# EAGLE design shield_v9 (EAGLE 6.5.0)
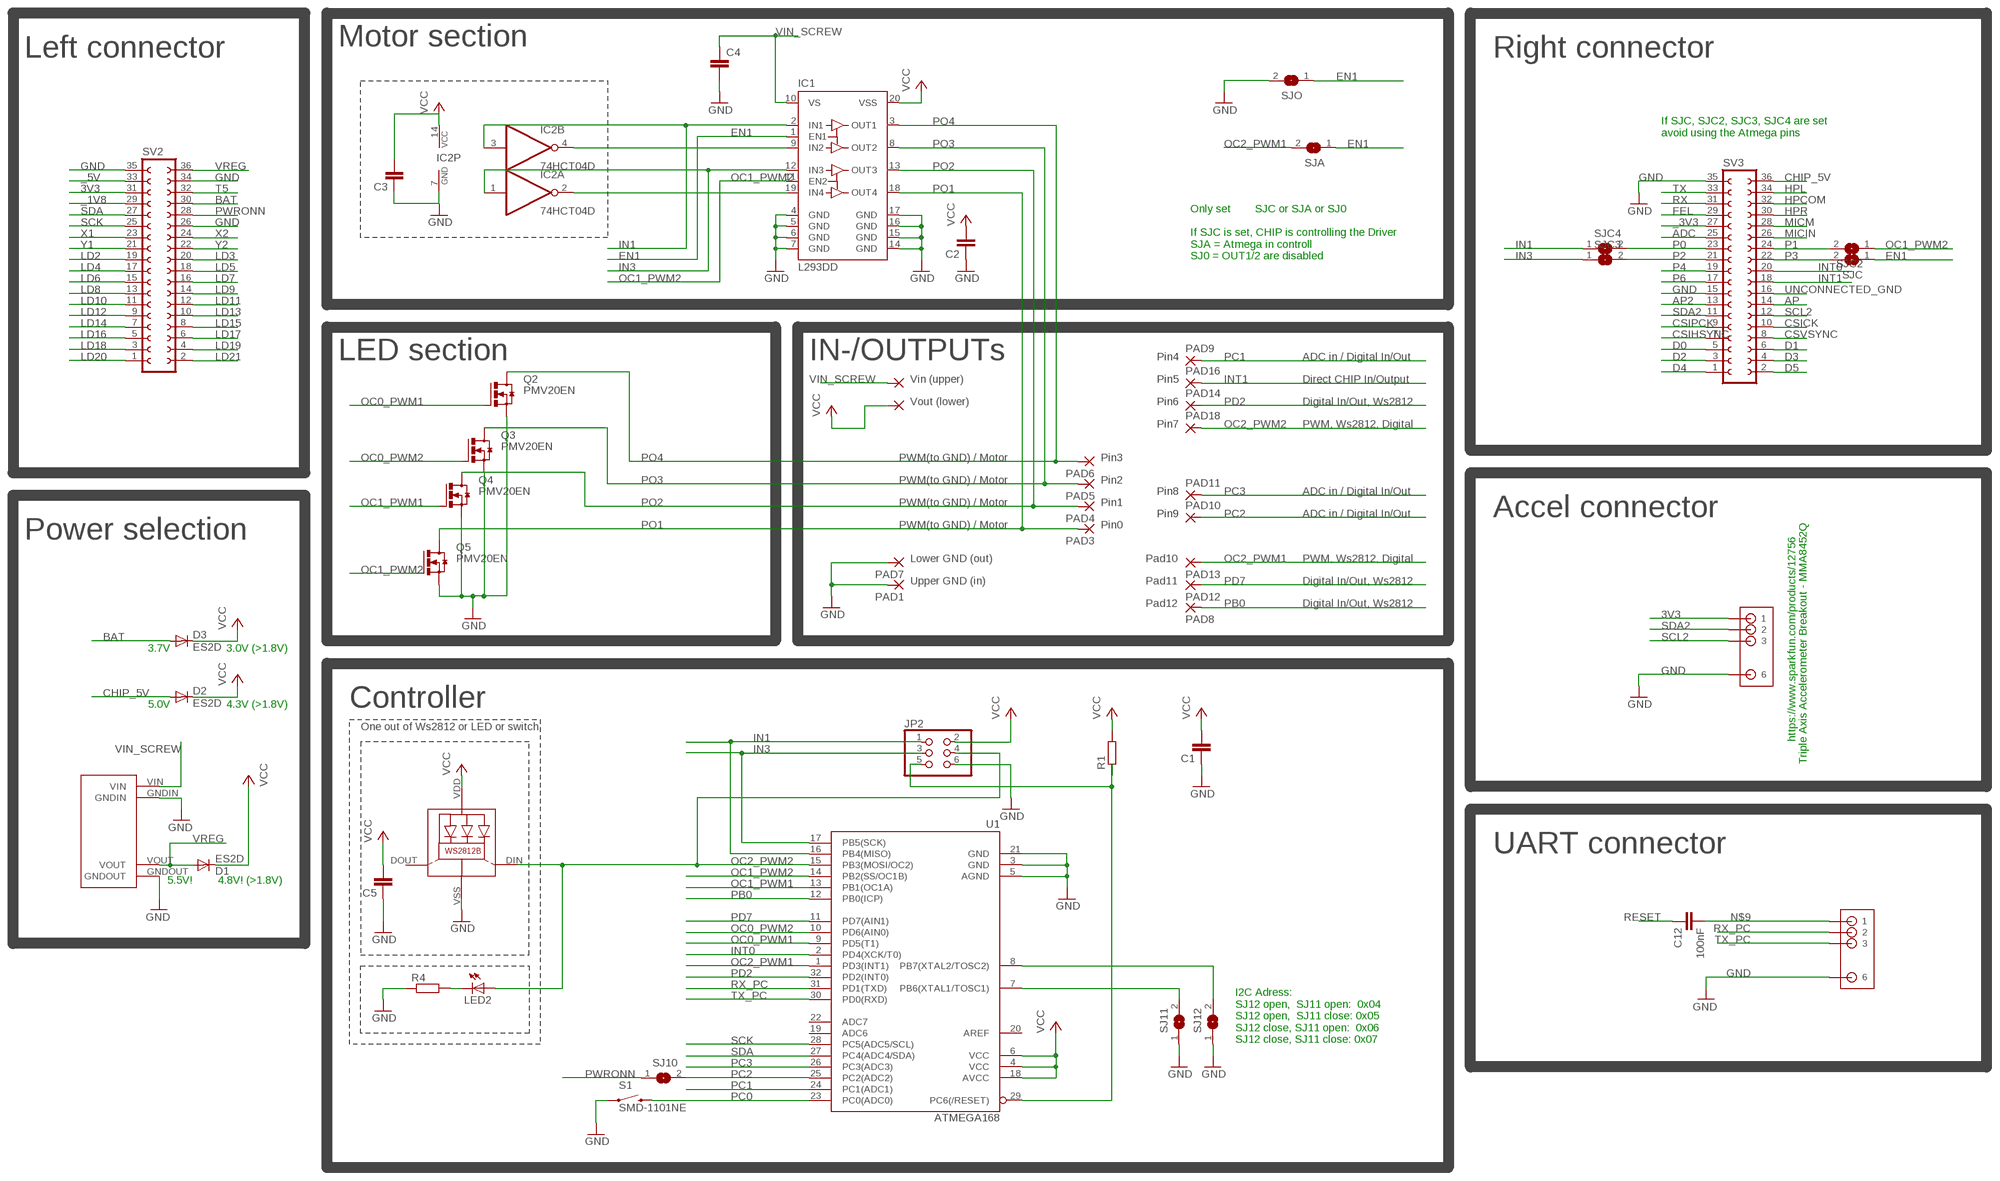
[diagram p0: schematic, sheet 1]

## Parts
C1  C-EUC0805  [C0805]
C2  C-EUC0805  [C0805]
C3  C-EUC0805  [C0805]
C4  C-EUC1210  [C1210]
C5  C-EUC0805  [C0805]
C12  100nF  C-EUC1206  [C1206]
D1  ES2D  [SMB]
D2  ES2D  [SMB]
D3  ES2D  [SMB]
IC1  L293DD  [SO20]
IC2  74HCT04D  [SO14]
JP2  PINHD-2X3  [2X03]
LED1  WS2812B  [WS2812B]
LED2  LEDCHIP-LED0805  [CHIP-LED0805]
PAD1  3,17/1,3  [3,17/1,3]
PAD2  3,17/1,3  [3,17/1,3]
PAD3  3,17/1,3  [3,17/1,3]
PAD4  3,17/1,3  [3,17/1,3]
PAD5  3,17/1,3  [3,17/1,3]
PAD6  3,17/1,3  [3,17/1,3]
PAD7  3,17/1,3  [3,17/1,3]
PAD8  WIREPADSMD1,27-254  [SMD1,27-2,54]
PAD9  3,17/1,3  [3,17/1,3]
PAD10  3,17/1,3  [3,17/1,3]
PAD11  3,17/1,3  [3,17/1,3]
PAD12  SMD2  [SMD1,27-2,54]
PAD13  SMD2  [SMD1,27-2,54]
PAD14  3,17/1,3  [3,17/1,3]
PAD16  3,17/1,3  [3,17/1,3]
PAD17  3,17/1,3  [3,17/1,3]
PAD18  3,17/1,3  [3,17/1,3]
Q2  PMV20EN  NMOSFET_SMD_223  [SOT223]
Q3  PMV20EN  NMOSFET_SMD_223  [SOT223]
Q4  PMV20EN  NMOSFET_SMD_223  [SOT223]
Q5  PMV20EN  NMOSFET_SMD_223  [SOT223]
R1  R-EU_M1206  [M1206]
R4  R-EU_M1206  [M1206]
S1  SMD-1101NE  SWITCH-MOMENTARY-2-SMD-1101NE  [TACTILE-SWITCH-1101NE]
SJ10  SJ  [SJ]
SJ11  SJ  [SJ]
SJ12  SJ  [SJ]
SJA  SJ  [SJ]
SJC  SJ  [SJ]
SJC2  SJ  [SJ]
SJC3  SJ  [SJ]
SJC4  SJ  [SJ]
SJO  SJ  [SJ]
SV2  FE18-2  [FE18-2]
SV3  FE18-2  [FE18-2]
U1  ATMEGA168  [TQFP32-08]
U$1  MP1584EN  [MP1584EN]
U$3  6_TO_4_HEADER  [6_TO_4_HEADER]
U$4  6_TO_4_HEADER  [6_TO_4_HEADER]

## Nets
3V3: SV2.31 U$4.1
_1V8: SV2.29
_3V3: SV3.27
_5V: SV2.33
ADC: SV3.25
AP: SV3.14
AP2: SV3.13
BAT: D3.A SV2.30
CHIP_5V: D2.A SV3.36
CSICK: SV3.10
CSIHSYNC: SV3.7
CSIPCK: SV3.9
CSVSYNC: SV3.8
D0: SV3.5
D1: SV3.6
D2: SV3.3
D3: SV3.4
D4: SV3.1
D5: SV3.2
EN1: IC1.1(EN1) SJA.1 SJC.1 SJO.1
FEL: SV3.29
GND: C1.1 C2.1 C3.1 C4.2 C5.1 IC1.4(GND) IC1.5(GND) IC1.6(GND) IC1.7(GND) IC1.14(GND) IC1.15(GND) IC1.16(GND) IC1.17(GND) IC2.7(P:GND) JP2.6 LED1.VSS(GND) PAD1.1(P) PAD7.1(P) Q2.3(S) Q3.3(S) Q4.3(S) Q5.3(S) R4.1 S1.P$1 SJ11.1 SJ12.1 SJO.2 SV2.26 SV2.34 SV2.35 SV3.15 SV3.35 U1.3(GND) U1.5(AGND) U1.21(GND) U$1.GNDIN U$1.GNDOUT U$3.6 U$4.6
HPCOM: SV3.32
HPL: SV3.34
HPR: SV3.30
IN1: IC1.2(IN1) IC2.3(B:I) JP2.1 SJC4.1 U1.16(PB4(MISO))
IN3: IC1.12(IN3) IC2.1(A:I) JP2.3 SJC3.1 U1.17(PB5(SCK))
INT0: SV3.20 U1.2(PD4(XCK/T0))
INT1: PAD16.1(P) SV3.18
LD2: SV2.19
LD3: SV2.20
LD4: SV2.17
LD5: SV2.18
LD6: SV2.15
LD7: SV2.16
LD8: SV2.13
LD9: SV2.14
LD10: SV2.11
LD11: SV2.12
LD12: SV2.9
LD13: SV2.10
LD14: SV2.7
LD15: SV2.8
LD16: SV2.5
LD17: SV2.6
LD18: SV2.3
LD19: SV2.4
LD20: SV2.1
LD21: SV2.2
MICIN: SV3.26
MICM: SV3.28
N$1: IC1.19(IN4) IC2.2(A:O)
N$2: SJ11.2 U1.7(PB6(XTAL1/TOSC1))
N$3: SJ12.2 U1.8(PB7(XTAL2/TOSC2))
N$4: LED2.C R4.2
N$9: C12.2 U$3.1
N$11: IC1.9(IN2) IC2.4(B:O)
OC0_PWM1: Q2.1(G) U1.9(PD5(T1))
OC0_PWM2: Q3.1(G) U1.10(PD6(AIN0))
OC1_PWM1: Q4.1(G) U1.13(PB1(OC1A))
OC1_PWM2: IC1.11(EN2) Q5.1(G) SJC2.1 U1.14(PB2(SS/OC1B))
OC2_PWM1: PAD13.1(P) SJA.2 U1.1(PD3(INT1))
OC2_PWM2: JP2.4 LED1.DIN(DI) LED2.A PAD18.1(P) U1.15(PB3(MOSI/OC2))
P0: SJC4.2 SV3.23
P1: SJC2.2 SV3.24
P2: SJC3.2 SV3.21
P3: SJC.2 SV3.22
P4: SV3.19
P6: SV3.17
PB0: PAD8.1(P) U1.12(PB0(ICP))
PC0: S1.P$2 U1.23(PC0(ADC0))
PC1: PAD9.1(P) U1.24(PC1(ADC1))
PC2: PAD10.1(P) SJ10.2 U1.25(PC2(ADC2))
PC3: PAD11.1(P) U1.26(PC3(ADC3))
PD2: PAD14.1(P) U1.32(PD2(INT0))
PD7: PAD12.1(P) U1.11(PD7(AIN1))
PO1: IC1.18(OUT4) PAD3.1(P) Q5.2(D) Q5.4(D)
PO2: IC1.13(OUT3) PAD4.1(P) Q4.2(D) Q4.4(D)
PO3: IC1.8(OUT2) PAD5.1(P) Q3.2(D) Q3.4(D)
PO4: IC1.3(OUT1) PAD6.1(P) Q2.2(D) Q2.4(D)
PWRONN: SJ10.1 SV2.28
RESET: C12.1 JP2.5 R1.1 U1.29(PC6(/RESET))
RX: SV3.31
RX_PC: U1.31(PD1(TXD)) U$3.2
SCK: SV2.25 U1.28(PC5(ADC5/SCL))
SCL2: SV3.12 U$4.3
SDA: SV2.27 U1.27(PC4(ADC4/SDA))
SDA2: SV3.11 U$4.2
T5: SV2.32
TX: SV3.33
TX_PC: U1.30(PD0(RXD)) U$3.3
UNCONNECTED_GND: SV3.16
VCC: C1.2 C2.2 C3.2 C5.2 D1.C D2.C D3.C IC1.20(VSS) IC2.14(P:VCC) JP2.2 LED1.VDD PAD17.1(P) R1.2 U1.4(VCC) U1.6(VCC) U1.18(AVCC)
VIN_SCREW: C4.1 IC1.10(VS) PAD2.1(P) U$1.VIN
VREG: D1.A SV2.36 U$1.VOUT
X1: SV2.23
X2: SV2.24
Y1: SV2.21
Y2: SV2.22
Unconnected: IC2.5(C:I) IC2.6(C:O) IC2.8(D:O) IC2.9(D:I) IC2.10(E:O) IC2.11(E:I) IC2.12(F:O) IC2.13(F:I) LED1.DOUT(DO) U1.19(ADC6) U1.20(AREF) U1.22(ADC7)

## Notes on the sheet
- Motor section
- Left connector | Right connector
- If SJC, SJC2, SJC3, SJC4 are set 
  avoid using the Atmega pins
- Only set        SJC or SJA or SJ0
  
  If SJC is set, CHIP is controlling the Driver
  SJA = Atmega in controll
  SJ0 = OUT1/2 are disabled
- LED section | IN-/OUTPUTs | Pin4 | ADC in / Digital In/Out
- Vin (upper) | Pin5 | Direct CHIP In/Output
- Vout (lower) | Pin6 | Digital In/Out, Ws2812
- Pin7 | PWM, Ws2812, Digital
- PWM(to GND) / Motor | Pin3
- PWM(to GND) / Motor | Pin2
- Pin8 | ADC in / Digital In/Out
- PWM(to GND) / Motor | Pin1
- Pin9 | ADC in / Digital In/Out | Accel connector
- PWM(to GND) / Motor | Pin0
- Power selection
- Lower GND (out) | Pad10 | PWM, Ws2812, Digital
- Upper GND (in) | Pad11 | Digital In/Out, Ws2812
- Pad12 | Digital In/Out, Ws2812
- 3.7V | 3.0V (>1.8V)
- 5.0V | 4.3V (>1.8V) | Controller
- One out of Ws2812 or LED or switch
- https://www.sparkfun.com/products/12756
- Triple Axis Accelerometer Breakout - MMA8452Q
- UART connector
- 5.5V! | 4.8V! (>1.8V)
- I2C Adress: 
  SJ12 open,  SJ11 open:  0x04
  SJ12 open,  SJ11 close: 0x05
  SJ12 close, SJ11 open:  0x06
  SJ12 close, SJ11 close: 0x07

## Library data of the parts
C1-C5 C12 = rcl:C-EU: CAPACITOR, European symbol
D1-D3 = diode:ES2D: DIODE
IC1 = st-microelectronics:L293DD: PUSH-PULL FOUR CHANNEL DRIVER WITH DIODES Source: http://www.st.com/stonline/books/pdf/docs/1330.pdf; OC_FARNELL: unknown
IC2 = 74xx-eu:74*04: Hex INVERTER
JP2 = pinhead:PINHD-2X3: PIN HEADER
LED1 = WS2812B:WS2812B: Features and Benefits  * Intelligent reverse connect protection, the power supply reverse connection does not damage the IC. * The control circuit and the LED share the only power source. Control circuit and RGB chip are integrated in a package of 5050 components, form a complete control of pixel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
LED2 = led:LED: LED
PAD1-PAD7 PAD9-PAD11 PAD14 PAD16-PAD18 = wirepad:3,17/1,3: THROUGH-HOLE PAD
PAD8 = wirepad:WIREPAD: Wire PAD connect wire on PCB
PAD12 PAD13 = wirepad:SMD2: SMD PAD
Q2-Q5 = transistor-power:NMOSFET_SMD_223
R1 R4 = rcl:R-EU_: RESISTOR, European symbol
S1 = SparkFun-Electromechanical:SWITCH-MOMENTARY-2: Various NO switches- pushbuttons, reed, etc
SJ10-SJ12 SJA SJC SJC2-SJC4 SJO = jumper:SJ: SMD solder JUMPER
SV2 SV3 = con-lsta:FE18-2: FEMALE HEADER; OC_FARNELL: unknown; OC_NEWARK: unknown
U1 = SparkFun-DigitalIC:ATMEGA168: Atmel 32-pin 8-bit micro, 16k flash.
U$1 = power_supply:MP1584EN
U$3 U$4 = power_supply:6_TO_4_HEADER

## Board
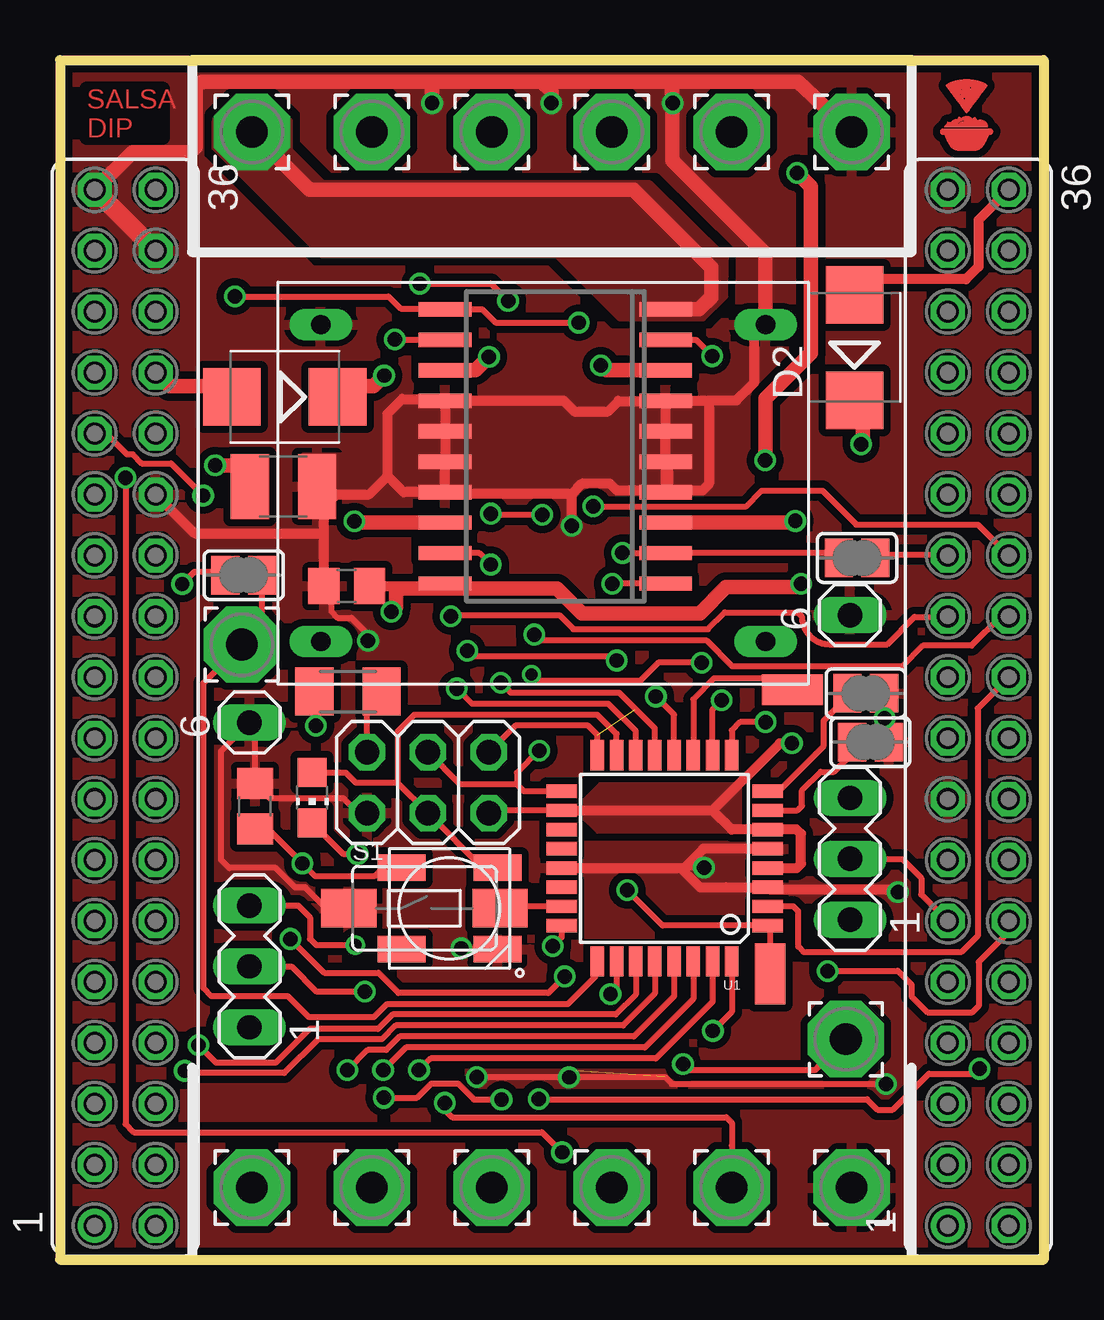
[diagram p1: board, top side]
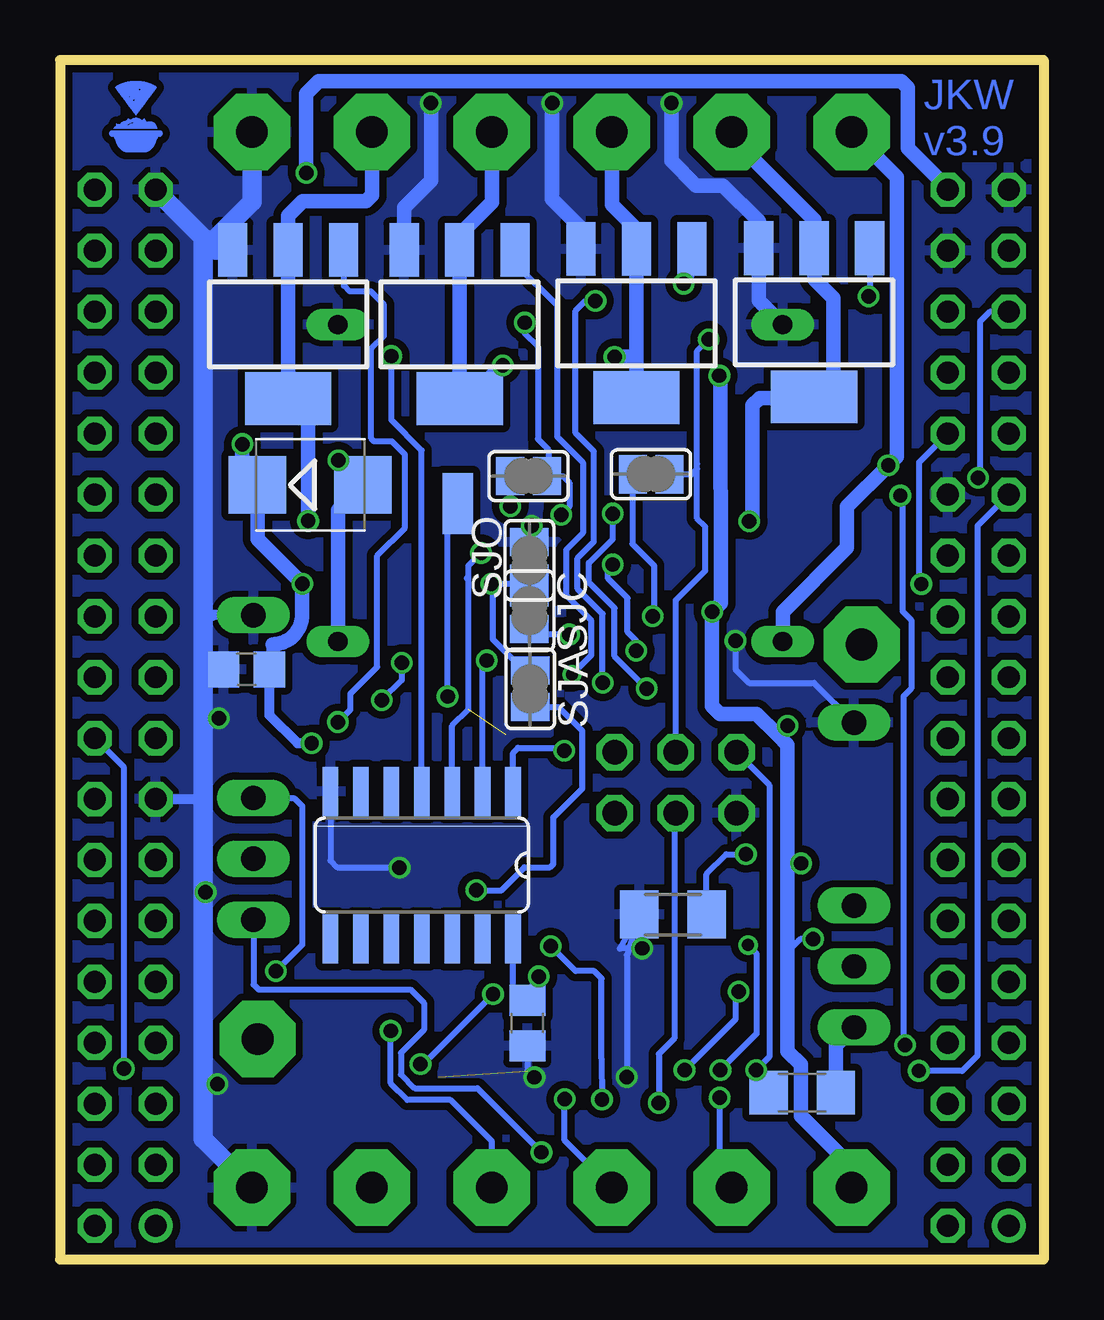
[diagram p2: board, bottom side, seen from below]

Size 41 x 50 mm. Coordinates in mm from the lower left corner, seen from the top.
Outline: 0,50 41,50 41,0 0,0 0,50
Copper layers (1*16): Top 0.035mm / dielectric 1.5mm / Bottom 0.035mm
Design rules "SeeedStudio_2layer_DRU_no_angle_20140221": minimum track width 6mil, minimum drill 12mil, track to track 6mil, track to pad 6mil, pad to pad 6mil, via to via 6mil, smd to smd 0mil, copper to edge 10mil, drill to drill 10mil, minimum pad ring 10mil, minimum via ring 6mil, stop-mask expansion 2mil, vias tented up to drill 100mil, thermal gap 10mil

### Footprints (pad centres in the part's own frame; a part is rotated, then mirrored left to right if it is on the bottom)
C0805 = smd 1.3 x 1.5: 1 -0.95,0; 2 0.95,0
C1210 = smd 1.6 x 2.7: 1 -1.4,0; 2 1.4,0
C1206 = smd 1.6 x 1.8: 1 -1.4,0; 2 1.4,0
SMB = smd 2.4 x 2.4: A 2.2,0; C -2.2,0
SO20 = smd 0.6 x 2.2: 1 -5.715,-4.6; 2 -4.445,-4.6; 3 -3.175,-4.6; 4 -1.905,-4.6; 5 -0.635,-4.6; 6 0.635,-4.6; 7 1.905,-4.6; 8 3.175,-4.6; 9 4.445,-4.6; 10 5.715,-4.6; 11 5.715,4.6; 12 4.445,4.6; 13 3.175,4.6; 14 1.905,4.6; 15 0.635,4.6; 16 -0.635,4.6; 17 -1.905,4.6; 18 -3.175,4.6; 19 -4.445,4.6; 20 -5.715,4.6
SO14 = smd 0.66 x 2.032: 1 -3.81,-3.073; 2 -2.54,-3.073; 3 -1.27,-3.073; 4 0,-3.073; 5 1.27,-3.073; 6 2.54,-3.073; 7 3.81,-3.073; 8 3.81,3.073; 9 2.54,3.073; 10 1.27,3.073; 11 0,3.073; 12 -1.27,3.073; 13 -2.54,3.073; 14 -3.81,3.073
2X03 = drill 1.016 octagon: 1 -2.54,-1.27; 2 -2.54,1.27; 3 0,-1.27; 4 0,1.27; 5 2.54,-1.27; 6 2.54,1.27
WS2812B = smd 2 x 1.1: DIN 2,1.7; DOUT -2,-1.7; VDD -2,1.7; VSS 2,-1.7
CHIP-LED0805 = smd 1.2 x 1.2: A 0,-1.05; C 0,1.05
3,17/1,3 = drill 1.321 pad 3.175 octagon: 1 0,0
SMD1,27-2,54 = smd 1.27 x 2.54: 1 0,0
SOT223 = smd 1.219 x 2.235: 1 -2.311,-3.099; 2 0,-3.099; 3 2.311,-3.099 | smd 3.6 x 2.2: 4 0,3.099
M1206 = smd 1.6 x 2: 1 -1.4,0; 2 1.4,0
TACTILE-SWITCH-1101NE = smd 2.3 x 1.6: P$1 -3.15,0; P$2 3.15,0
SJ = smd 1.168 x 1.6: 1 -0.762,0; 2 0.762,0
FE18-2 = drill 0.914: 1 -21.59,1.27 | drill 0.914 octagon: 2 -21.59,-1.27; 3 -19.05,1.27; 4 -19.05,-1.27; 5 -16.51,1.27; 6 -16.51,-1.27; 7 -13.97,1.27; 8 -13.97,-1.27; 9 -11.43,1.27; 10 -11.43,-1.27; 11 -8.89,1.27; 12 -8.89,-1.27; 13 -6.35,1.27; 14 -6.35,-1.27; 15 -3.81,1.27; 16 -3.81,-1.27; 17 -1.27,1.27; 18 -1.27,-1.27; 19 1.27,1.27; 20 1.27,-1.27; 21 3.81,1.27; 22 3.81,-1.27; 23 6.35,1.27; 24 6.35,-1.27; 25 8.89,1.27; 26 8.89,-1.27; 27 11.43,1.27; 28 11.43,-1.27; 29 13.97,1.27; 30 13.97,-1.27; 31 16.51,1.27; 32 16.51,-1.27; 33 19.05,1.27; 34 19.05,-1.27; 35 21.59,1.27; 36 21.59,-1.27
TQFP32-08 = smd 1.27 x 0.559: 1 -4.293,2.8; 2 -4.293,2; 3 -4.293,1.2; 4 -4.293,0.4; 5 -4.293,-0.4; 6 -4.293,-1.2; 7 -4.293,-2; 8 -4.293,-2.8; 17 4.293,-2.8; 18 4.293,-2; 19 4.293,-1.2; 20 4.293,-0.4; 21 4.293,0.4; 22 4.293,1.2; 23 4.293,2; 24 4.293,2.8 | smd 0.559 x 1.27: 9 -2.8,-4.293; 10 -2,-4.293; 11 -1.2,-4.293; 12 -0.4,-4.293; 13 0.4,-4.293; 14 1.2,-4.293; 15 2,-4.293; 16 2.8,-4.293; 25 2.8,4.293; 26 2,4.293; 27 1.2,4.293; 28 0.4,4.293; 29 -0.4,4.293; 30 -1.2,4.293; 31 -2,4.293; 32 -2.8,4.293
MP1584EN = drill 0.8 long: GNDIN 1.778,14.986; GNDOUT 20.32,14.986; VIN 1.778,1.778; VOUT 20.32,1.778
6_TO_4_HEADER = drill 1.016 long: 1 0,-6.35; 2 0,-3.81; 3 0,-1.27; 6 0,6.35

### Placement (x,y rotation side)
C1  33.22,24.6 0 bottom
C2  11.95,28.07 0 top
C3  21.52,9.85 90 bottom
C4  9.32,32.22 0 top
C5  8.13,18.9 270 top
C12  10.06,6.96 0 bottom
D1  30.57,32.28 0 bottom
D2  33.12,38.01 90 top
D3  9.37,35.95 180 top
IC1  20.65,33.89 90 top
IC2  25.92,16.44 180 bottom
JP2  15.34,19.88 180 top
LED1  16.23,14.63 0 top
LED2  10.52,19.25 180 top
PAD1  33,47 0 top
PAD2  8,47 0 top
PAD3  13,47 0 top
PAD4  18,47 0 top
PAD5  23,47 0 top
PAD6  28,47 0 top
PAD7  33,3 0 top
PAD8  24.42,31.5 180 bottom
PAD9  13,3 0 top
PAD10  7.58,25.63 0 top
PAD11  32.76,9.18 0 top
PAD12  30.52,23.76 270 top
PAD13  29.6,11.9 180 top
PAD14  23,3 0 top
PAD16  18,3 0 top
PAD17  8,3 0 top
PAD18  28,3 0 top
Q2  31.49,38.98 180 bottom
Q3  24.34,38.98 180 bottom
Q4  16.97,39.02 180 bottom
Q5  9.56,39.06 180 bottom
R1  12.01,23.67 180 top
R4  15.45,14.38 0 bottom
S1  15.19,14.64 0 top
SJ10  7.66,28.52 0 top
SJ11  33.78,21.56 180 top
SJ12  33.59,23.6 180 top
SJA  21.4,23.79 270 bottom
SJC  21.43,27.05 270 bottom
SJC2  21.47,32.66 180 bottom
SJC3  16.36,32.74 180 bottom
SJC4  33.23,29.24 0 top
SJO  21.43,29.15 90 bottom
SV2  2.72,23 90 top
SV3  38.28,23 90 top
U1  25.2,16.72 180 top
U$1  9.09,23.98 0 top
U$2  LOGO  [LOGO]  36.54,46.02 0 top
U$3  7.9,16.03 0 top
U$4  32.93,20.51 0 top
U$5  LOGO  [LOGO]  39.09,46.1 0 bottom

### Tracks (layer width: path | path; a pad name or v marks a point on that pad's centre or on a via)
3V3  (via drill 0.6)
  Top 0.254: v2.73,32.59 2.73,5.65 3.07,5.31 20.09,5.31 v20.93,4.47
  Bottom 0.254: U$4.1 32.93,11.47 32.72,11.25 26.39,11.25 25.83,10.69 25.83,9.56 26.78,8.61 26.78,7.71 26.21,7.14 23.6,7.14 v20.93,4.47 | SV2.31 2.23,39.51 2.65,39.09 2.65,32.66 v2.73,32.59
BAT
  Top 0.61: SV2.30 4.56,36.4 6.73,36.4 D3.A
CHIP_5V
  Top 0.406: SV3.36 38.29,43.33 38.29,41.38 37.77,40.86 34.13,40.86 D2.A
EN1  (via drill 0.6)
  Top 0.254: IC1.1 v23.03,28.18 v23.02,28.17
  Bottom 0.254: SJA.1 21.65,24.55 22.95,25.84 22.95,28.09 v23.02,28.17 21.65,28.17 SJO.1 SJC.1 21.2,28.18
  Bottom 0.406: 21.37,27.87 SJC.1
GND  (via drill 0.6)  (1 unrouted)
  Top 0.254: C5.1 8.13,22.15 U$3.6 6.72,21.2 6.72,16.66 7.06,16.32 8.99,16.32 9.79,15.52 10.22,15.52 11.1,14.64 S1.P$1 | v26.85,16.33 26.18,16.33 26.11,16.4 | 34.35,21.75 SJ11.1 34.38,21.73 v34.38,22.57 34.35,22.59 SJ12.1 | C2.1 11.3,27.77 11.3,27.03 11.58,26.75 12.15,26.75 12.84,26.06 v12.84,25.79 | LED1.VSS 16.76,12.93 v16.73,12.97 | v17.37,7.61 25.21,7.61 25.5,7.32 v34.44,7.32 | C5.1 | JP2.6 12.43,18.61 11.82,19.21 8.76,19.21 C5.1
  Top 0.406: U1.21 25.87,16.32 25.95,16.24 | 29.45,17.08 U1.5 26.82,17.12 26.11,16.4 25.95,16.24 | 27.77,15.52 U1.3 | 25.95,16.24 26.67,15.52 U1.3 | IC1.7 23.28,35.79 22.84,35.34 21.45,35.34 21,35.8 IC1.14 IC1.15 | IC1.7 27.03,35.8 27.05,35.81 | 27.05,35.81 27.05,32.32 26.78,32.05 25.32,32.05 | 25.32,32.05 IC1.4 | 25.32,32.05 23.22,32.05 22.94,32.33 21.77,32.33 21.35,31.91 | 21.35,31.91 16.12,31.91 IC1.17 | IC1.17 14.33,31.99 13.65,32.66 | 13.65,32.66 13.65,35.26 14.26,35.87 16,35.87 16.03,35.84 | 27.05,35.81 28.21,35.81 28.94,36.55 28.94,38.49 U$1.GNDOUT | IC1.17 IC1.16 | IC1.15 16.05,33.28 16.07,33.26 16.07,34.51 IC1.15 | IC1.7 25.24,32.09 25.38,31.95 25.38,33.13 IC1.5 IC1.6 | 13.65,32.66 12.88,31.89 11.53,31.89 11,31.36 11,30.26 | C2.1 11,30.26 | SV2.26 5.62,30.26 11,30.26 | U1.3 29.58,15.43 34.81,15.43 v34.93,15.31 | SJ11.1 34.51,21.6 | v21.34,30.58 21.34,31.9 21.35,31.91
  Top 0.61: 15.51,49.1 20.08,49.1 | 20.08,49.1 25.51,49.1 | 25.51,49.1 30.77,49.1 PAD1.1 | 25.51,49.1 25.51,48.52 v25.54,48.2 25.54,45.8 29.41,41.92 U$1.GNDOUT | v15.51,48.2 15.51,49.1 | v20.48,48.2 20.48,48.7 20.08,49.1 | 15.51,49.1 5.92,49.1 5.66,48.84 5.66,46.35 5.47,46.16 3.02,46.16 SV2.35
  Top 0.813: SV2.35 SV2.34
  Bottom 0.254: R4.1 17.37,12.68 v17.37,7.61 | 17.65,12.95 R4.1 | C3.1 21.52,7.87 v21.22,7.59 | 34.63,26.84 35.04,27.24 | IC2.7 29.73,16.63 29.44,16.34 26.86,16.34 v26.85,16.33 | C1.1 34.26,24.69 35.04,24.69 | 32.63,47.37 PAD1.1 | v12.84,25.79 12.84,24.6 12.28,24.04 9.56,24.04 U$3.6 | v16.73,12.97 17.66,12.97 R4.1
  Bottom 0.406: SV3.15 35.11,19.19 35.04,19.12 | 35.05,15.41 35.04,15.42 | 35.04,15.2 v34.93,15.31 34.93,15.71 35.04,15.82 | 35,21.45 35.04,21.41 | 34.92,21.43 34.9,21.45 35.04,21.59 35.04,21.61 | 34.89,26.55 35.04,26.4 | v34.44,7.32 35.04,7.32 | 34.84,38.95 35.04,38.75 | v34.38,22.57 34.56,22.49 35.04,22.02 | U$4.6 34.61,26.86 34.63,26.84 | SJO.2 21.37,30.54 v21.34,30.58
  Bottom 0.61: Q3.3 26.65,43.85 25.54,44.96 v25.54,48.2 | v15.51,48.2 15.51,45.8 14.48,44.77 13.36,44.77 11.87,43.28 Q5.3 11.87,39.96 U$1.GNDIN | Q4.3 19.28,42.99 20.49,44.2 20.48,44.21 v20.48,48.2
  Bottom 0.813: 35.04,42.6 35.04,38.75 35.04,27.24 35.04,26.4 35.04,24.69 35.04,22.02 35.04,21.61 35.04,21.41 35.04,19.12 35.04,15.82 35.04,15.42 35.04,15.2 35.04,7.32 35.04,5.04 PAD7.1 | Q2.3 34.52,42.08 34.76,42.33 | 34.76,42.33 35.04,42.6 | PAD1.1 33,44.09 34.76,42.33 | SV3.35 37.01,44.57 35.04,42.6
  pour Top (isolate 0.305, rank 2): -0.07,0.25 40.88,0.25 41.01,10.57 41.01,50.01 0,50.01 0,10.47
  pour Bottom (isolate 0.305): 0,50 41.05,50 41.05,0.25 0.02,0.25 0.02,49.92
  pour Top (isolate 0.305, no thermals): 13.28,33.52 14.05,35.84 20.97,35.9 21.42,35.45 22.83,35.45 23.2,35.81 28.13,35.81 28.24,35.7 28.24,32.35 27.85,31.95 23.33,31.95 23.05,32.23 21.77,32.23 21.4,31.86 11.16,31.85 10.36,32.65 10.15,33.49
IN1  (via drill 0.6)  (1 unrouted)
  Top 0.254: JP2.1 18.98,22.25 22.02,22.25 22.4,21.87 U1.16 | v23.44,29.45 IC1.2 32.26,29.45 SJC4.1
  Bottom 0.254: IC2.3 24.65,22.25 23.98,22.92 23.98,28.46 | 23.98,28.46 23.98,28.92 v23.44,29.45 | 24.04,28.4 23.98,28.46
IN3  (via drill 0.6)
  Top 0.254: U1.17 19.34,19.52 19.05,19.81 | 19.05,19.81 16.68,19.81 JP2.3 | v19.98,21.21 19.05,20.28 19.05,19.81 | v13.96,38.35 16.03,38.35 IC1.12
  Bottom 0.254: JP2.3 15.34,27.47 14.1,28.71 14.1,30.54 14.44,30.89 14.44,32.96 | IC2.1 22.11,21.12 21.91,21.32 20.09,21.32 v19.98,21.21 | 14.22,38.09 v13.96,38.35 14.44,37.87 14.44,33.16 14.44,32.96 | SJC3.1 14.66,32.73 14.44,32.96
INT0
  Top 0.254: SV3.20 38.25,22.97 38.25,13.49 37.59,12.83 30.99,12.83 30.77,13.04 30.77,14.52 30.57,14.72 U1.2
INT1  (via drill 0.6)
  Top 0.254: v38.33,7.95 38.13,7.75 36.22,7.75 34.72,6.25 34.07,6.25 33.64,6.68 v19.96,6.68
  Bottom 0.254: PAD16.1 19.96,4.96 v19.96,6.68 | v38.33,7.95 38.33,20.51 SV3.18
N$1  (via drill 0.6)
  Top 0.254: 17.21,25.15 v16.98,25.38 17.22,25.13 23.04,25.13 v23.2,24.97 | v17.96,28.97 17.48,29.45 IC1.19
  Bottom 0.254: IC2.2 23.38,24.83 23.34,24.83 v23.2,24.97 | v16.98,25.38 16.98,25.79 17.34,26.15 17.34,27.57 18.15,28.38 18.15,28.78 v17.96,28.97
N$2
  Top 0.254: U1.7 30.75,18.72 30.94,18.91 30.94,19.56 31.71,20.33 32.27,20.33 33.03,21.09 33.03,21.78 33.03,22.12
  Top 0.406: SJ11.2 33.03,21.58 33.03,21.78
N$3
  Top 0.254: U1.8 29.95,19.52 31.84,21.41 31.84,22.47 32.83,23.46 SJ12.2
N$4  (via drill 0.6)
  Top 0.254: LED2.C 11.82,16.89 v12.41,16.89
  Bottom 0.254: R4.2 14.05,16.06 13.22,16.89 v12.41,16.89
N$9
  Bottom 0.406: 7.9,9.61 U$3.1
  Bottom 0.61: C12.2 8.66,8.92 U$3.1
N$11  (via drill 0.6)
  Top 0.254: IC1.9 26.51,38.34 v27.19,37.66
  Bottom 0.254: IC2.4 25.92,33.73 27.19,35 v27.19,37.66
OC0_PWM1  (via drill 0.6)
  Top 0.254: v29.41,22.4 28.35,22.4 28,22.06 U1.9
  Bottom 0.254: v29.41,22.4 28.89,22.93 28.89,23.59 27.77,24.7 27.77,29.34 26.62,30.49 26.62,33.55 27.16,34.1 27.9,34.1 28.03,34.23 28.03,37.96 27.5,38.49 27.5,39.8 28.04,40.35 28.92,40.35 29.16,40.59 29.16,41.4 29.18,41.42 | 29.13,42.03 Q2.1
  Bottom 0.406: 29.18,41.42 Q2.1
OC0_PWM2  (via drill 0.5, 0.6)
  Top 0.254: U1.10 27.2,22.93 v27.58,23.32 | v19.66,24.38 19.91,24.13 24.19,24.13 24.94,24.88 v26.75,24.88
  Bottom 0.254: 22.1,42.01 Q3.1 22.03,41.51 20.27,39.75 20.27,34.29 19.2,33.22 19.2,30.28 19.89,29.59 19.89,27.67 18.85,26.63 18.85,25.2 v19.66,24.38 | v27.58,23.32 26.75,24.16 v26.75,24.88
  Bottom 0.406: Q3.1 22.06,42.05
OC1_PWM1  (via drill 0.6)
  Top 0.254: U1.13 24.8,22.14 23.32,23.62 18.8,23.62 v18.38,24.04 | v15,40.68 17.96,40.68 v18.68,39.96
  Bottom 0.254: v18.68,39.96 19.09,39.96 19.51,39.54 19.51,34.44 18.75,33.68 18.75,29.92 19.42,29.25 19.42,27.95 18.38,26.91 v18.38,24.04 | Q4.1 14.66,41.02 v15,40.68
OC1_PWM2  (via drill 0.6)
  Top 0.254: U1.14 24,22.02 22.86,23.16 17.18,23.16 v16.54,23.8 | v7.29,40.15 13.69,40.15 14.2,39.64 16.02,39.64 IC1.11 17.59,39.61 18.15,39.05 v21.63,39.05 | v20.1,31.04 18.01,31.04 v17.96,31.09
  Bottom 0.254: v16.54,23.8 17.88,25.14 17.88,27.15 18.95,28.22 18.95,29.03 17.96,30.02 v17.96,31.09 17.88,31.01 | Q5.1 7.25,40.19 v7.29,40.15 | v21.63,39.05 21.63,38.59 21.08,38.05 21.08,34.2 20.64,33.76 20.64,32.72 SJC2.1 20.03,32.66 19.76,32.38 19.76,31.38 v20.1,31.04
  Bottom 0.406: 7.25,42.99 Q5.1
OC2_PWM1  (via drill 0.6)
  Top 0.254: v23.65,15.39 25.12,13.92 U1.1 29.6,13.81 PAD13.1
  Bottom 0.254: v23.65,15.39 22.59,15.39 21.64,16.34 20.57,16.34 20.43,16.48 20.43,18.43 19.23,19.63 19.23,22.04 20.21,23.01 21.39,23.01 SJA.2
OC2_PWM2  (via drill 0.6)
  Top 0.254: PAD18.1 28,4.75 28,5.7 27.77,5.93 16.34,5.93 16.04,6.24 v16.04,6.53 | U1.15 23.2,21.91 22.4,22.71 14.77,22.71 14.08,22.02 14.08,19.87 | 14.08,19.87 JP2.4 17.62,16.33 LED1.DIN | LED2.A 11.91,20.3 12.33,19.88 14.07,19.88 14.08,19.87
  Bottom 0.254: JP2.4 15.39,18.56 15.39,9.22 16.04,8.57 v16.04,6.53
P0
  Top 0.254: SJC4.2 34.12,29.38 36.98,29.38
  Top 0.406: 36.98,29.38 SV3.23
P1  (via drill 0.6)
  Top 0.254: SV3.24 38.27,30.63 33.2,30.63 31.79,32.04 29.25,32.04 28.6,31.39 v22.23,31.39
  Bottom 0.254: v22.23,31.39 SJC2.2
P2  (via drill 0.6)
  Top 0.254: v16.29,26.81 16.34,26.86 20.82,26.86 21.4,26.28 27.01,26.28 27.71,26.98 30.76,26.98 30.92,26.81 arc90 32.09,25.64 34.48,25.64 35.62,26.78 36.98,26.78 SV3.21
  Bottom 0.254: 17.16,32.7 17.14,32.71 | 17.14,32.71 SJC3.2 | 17.14,32.71 17.14,29.83 16.23,28.92 16.23,26.87 v16.29,26.81
P3  (via drill 0.6)
  Top 0.254: SV3.22 39.22,26.81 38,25.59 35.98,25.59 35.12,24.73 28.03,24.73 26.96,25.79 20.03,25.79 v19.77,26.05
  Bottom 0.254: v19.77,26.05 21.2,26.05 SJC.2
PB0  (via drill 0.6)
  Top 0.254: U1.12 25.6,22.71 v24.84,23.47
  Bottom 0.254: v24.84,23.47 24.84,31.09 PAD8.1
PC0
  Top 0.254: U1.23 18.42,14.72 S1.P$2
PC1  (via drill 0.6)
  Top 0.254: v13.5,6.74 14.88,6.74 15.48,7.34 16.59,7.34 17.26,6.67 v18.41,6.67 | U1.24 20.91,13.43 v20.55,13.06
  Bottom 0.254: v18.41,6.67 18.42,8.36 18.42,11.71 18.73,12.03 19.51,12.03 v20.55,13.06 | v13.5,6.74 13.5,3.5 PAD9.1
PC2
  Top 0.254: SJ10.2 8.42,26.34 8.28,26.34 PAD10.1 5.98,24.04 5.98,11.32 6.31,10.99 9.5,10.99 10.39,10.1 13.08,10.1 13.64,10.65 21.17,10.65 22.34,11.82 22.34,12.37 U1.25
PC3  (via drill 0.6)
  Top 0.254: 31.57,8 PAD11.1 31.46,7.89 26.23,7.89 v25.97,8.14 | U1.26 23.2,11.31 v22.95,11.06
  Bottom 0.254: v22.95,11.06 25.87,8.14 v25.97,8.14
PD2  (via drill 0.6)
  Top 0.254: U1.32 28,10.31 v27.22,9.53
  Bottom 0.254: PAD14.1 23,4.93 24.73,6.66 26.52,6.66 27.22,7.35 v27.22,9.53
PD7
  Top 0.254: U1.11 26.4,23.35 27.28,24.23 30.05,24.23 PAD12.1
PO1  (via drill 0.6)
  Top 0.61: IC1.18 12.32,30.72 arc-90 v12.27,30.77
  Bottom 0.406: 9.38,35.78 Q5.4
  Bottom 0.61: PAD3.1 13,46.77 9.56,43.33 Q5.2 9.56,40.87 8.76,40.07 8.76,36.76 Q5.4 | 9.28,35.69 Q5.4 | Q5.4 9.61,35.92 11.82,35.92 12.13,35.61 12.13,30.91 v12.27,30.77
PO2  (via drill 0.6)
  Top 0.61: IC1.13 17.32,37.07 v17.88,37.63
  Bottom 0.61: PAD4.1 18,43.97 16.97,42.94 Q4.2 16.97,37.63 | 15.76,35.92 Q4.4 16.97,37.63 | v17.88,37.63 16.97,37.63
PO3  (via drill 0.6)
  Top 0.61: IC1.8 22.75,37.07 v22.54,37.27
  Bottom 0.61: PAD5.1 23,44.07 24.34,42.73 Q3.2 Q3.4 23.9,36.32 23.5,36.32 v22.54,37.27
PO4  (via drill 0.6)
  Top 0.61: IC1.3 30.59,30.72 v30.66,30.79
  Bottom 0.61: PAD6.1 28,44.37 28.25,44.12 30.88,44.12 31.49,43.51 Q2.2 Q2.4 30.82,35.21 30.66,35.05 v30.66,30.79
PWRONN  (via drill 0.6)
  Top 0.254: SJ10.1 6.76,28.66 5.6,28.66 v5.09,28.16
  Bottom 0.254: SV2.28 5.18,33.24 5.18,28.25 v5.09,28.16
RESET  (via drill 0.6)
  Top 0.254: U1.29 25.6,10.97 23.93,9.3 14.16,9.3 13.6,8.74 12.82,8.74 v11.98,7.89 11.98,7.94 | JP2.5 12.8,23.06 R1.1
  Bottom 0.254: C12.1 10.82,6.73 v11.98,7.89 11.43,8.44 11.43,19.78 JP2.5
  Bottom 0.406: 11.96,7.92 v11.98,7.89
RX_PC  (via drill 0.6)
  Top 0.254: U1.31 27.2,10.74 24.84,8.38 15.45,8.38 v14.96,7.89 | U$3.2 9.65,12.22 10.71,11.16 v12.71,11.16
  Bottom 0.254: v14.96,7.89 12.83,10.03 12.83,11.05 v12.71,11.16
SCK  (via drill 0.6)
  Top 0.254: U1.28 24.8,11.08 23.47,9.75 13.99,9.75 13.42,9.18 10.76,9.18 9.35,7.77 5.29,7.77 v5.2,7.86
  Bottom 0.254: v5.2,7.86 3.39,7.86 2.76,8.49 2.76,30.58 SV2.25
SCL2  (via drill 0.6)
  Top 0.254: 39.55,13.65 38.3,12.4 38.3,10.57 38.04,10.31 36.16,10.31 35.5,10.97 35.5,11.47 34.92,12.04 32.02,12.04 v32,12.02
  Top 0.406: SV3.12 39.55,13.65
  Bottom 0.254: v32,12.02 30.9,13.12 30.9,18.9 31.21,19.21 32.91,19.21 U$4.3
SDA  (via drill 0.6)
  Top 0.254: U1.27 24,11.05 23.16,10.21 13.86,10.21 13.26,9.61 10.4,9.61 8.99,8.2 6.5,8.2 v5.77,8.94 | v5.97,31.84 4.63,33.19 3.42,33.19 3.04,33.57 2.78,33.57 1.92,34.43 SV2.27
  Bottom 0.254: v5.97,31.84 5.88,31.75 5.88,27.03 5.51,26.66 5.51,23.8 5.84,23.47 5.84,9.02 v5.77,8.94
SDA2
  Top 0.254: SV3.11 35.9,15.21 35.9,15.9 35.13,16.68 32.96,16.68 U$4.2
TX_PC  (via drill 0.5, 0.6)
  Top 0.254: U1.30 26.4,10.86 24.38,8.84 14.42,8.84 v13.47,7.89 | U$3.3 9.93,14.76 10.43,14.26 10.43,13.36 10.68,13.11 v12.32,13.11
  Bottom 0.254: v13.47,7.89 v13.48,7.9 11.95,9.43 11.95,12.74 v12.32,13.11 12.04,12.83
VCC  (via drill 0.6)
  Top 0.254: U1.18 17.99,18.72 JP2.2 | 10.29,16.33 v10.11,16.51 | C5.2 8.67,17.95 v10.11,16.51 | R1.2 10.61,22.31 v10.67,22.25 | v33.4,33.98 33.48,34.06 | v9.6,13.36 11.01,11.95 13.27,11.95 14.11,11.11 20.36,11.11 v21.04,11.8 | LED1.VDD 13.46,16.33 13.11,15.98 10.64,15.98 v10.11,16.51
  Top 0.406: U1.18 27.2,18.72 | 27.2,18.72 30,21.52 v30.51,21.52 | C2.2 15.94,28.07 IC1.20 | D3.C 10.99,36.4 | U1.4 30.71,16.32 30.89,16.5 30.89,17.74 30.7,17.93 29.5,17.93 U1.6 28,17.92 27.2,18.72
  Top 0.61: 32.99,35.32 D2.C arc-90 33.48,35.46 33.48,34.06 | 15.84,27.96 14.02,27.96 14.02,27.2 v13.82,27 | 15.84,27.96 IC1.20 | 15.84,27.96 20.73,27.96 21.75,26.94 26.67,26.94 27.76,28.03 30.76,28.03 v30.9,28.17 | v13.51,36.84 13.07,36.4 11.27,36.4 11.16,36.3 11.23,36.3 D3.C
  Bottom 0.254: IC2.14 22.11,11.39 C3.2 21.27,11.05 21.27,11.57 v21.04,11.8 | v10.11,16.51 10.65,16.51 10.67,16.52 | 32.14,25.64 32.27,25.51 C1.2 | v10.67,22.25 10.72,22.25 11.09,21.88 | v9.6,13.36 10.13,13.36 10.67,12.83
  Bottom 0.406: 13.46,36.79 v13.51,36.84 | C1.2 32.27,22.7 31.1,21.53 v30.52,21.53 v30.51,21.52
  Bottom 0.61: v33.4,33.98 33.4,32.92 D1.C 32.77,30.04 v30.9,28.17 30.9,26.89 arc90 32.14,25.64 | PAD17.1 8,3.86 10.12,5.98 10.12,8.13 10.67,8.67 10.67,12.83 10.67,16.52 10.67,21.45 11.09,21.88 11.96,22.75 13.49,22.75 13.82,23.08 v13.82,27 13.45,27.37 13.46,36.79
  pour Top: 21.17,18.81 21.56,18.81 22.02,19.27 22.54,19.79 23.6,19.79 28.27,19.79 28.31,19.75 28.31,17.91 28.26,17.86 22.44,17.86 21.74,18.55 21.26,18.55 21.17,18.64
VIN_SCREW  (via drill 0.6)
  Top 0.61: IC1.10 26.64,39.61 27.15,40.12 27.15,41.35 23.9,44.6 10.4,44.6 PAD2.1 | C4.1 7.72,33.1 v6.47,33.1
  Bottom 0.61: PAD2.1 6.11,45.11 6.11,33.47 v6.47,33.1 8.19,31.38 8.19,29.67 10.87,26.99 U$1.VIN
  pour Top (isolate 0.254, no thermals): 6.43,47.37 6.43,46.35 10.92,41.86 20.7,41.86 23.33,39.23 26.82,39.23 27.74,40.14 27.76,41.74 24.6,44.86 10.95,44.89 9.6,46.24 9.6,47.45 8.69,48.36 7.33,48.36 6.45,47.49
VREG  (via drill 0.6)
  Top 0.61: v29.4,33.31 29.4,35.88 31.3,37.78 31.3,44.72 v30.73,45.29
  Bottom 0.254: D1.A v29.4,33.31
  Bottom 0.61: U$1.VOUT 29.41,31.24 D1.A | v30.73,45.29 30.73,48.59 30.21,49.11 5.92,49.11 5.65,48.84 5.65,46.32 3.99,44.66 SV2.36

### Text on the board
Top: SALSA / DIP
Bottom: JKW / v3.9
tStop: SALSA / DIP | SALSA DIP II v3.9 | 9 | 10 | 11 | 8: A_IN | 5V | 4:ADC | 5:C_IN | 6:A_IN | 7:NEO | GND
bStop: 5V | 0:PWM | 1:PWM | 2:PWM | 3:PWM | GND | JKW / v3.9 | 5V | 4:ADC | 5:C_IN | 7:NEO | GND | 6:A_IN

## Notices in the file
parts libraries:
SparkFun-DigitalIC: Licensing: Creative Commons ShareAlike 4.0 International - https://creativecommons.org/licenses/by-sa/4.0
